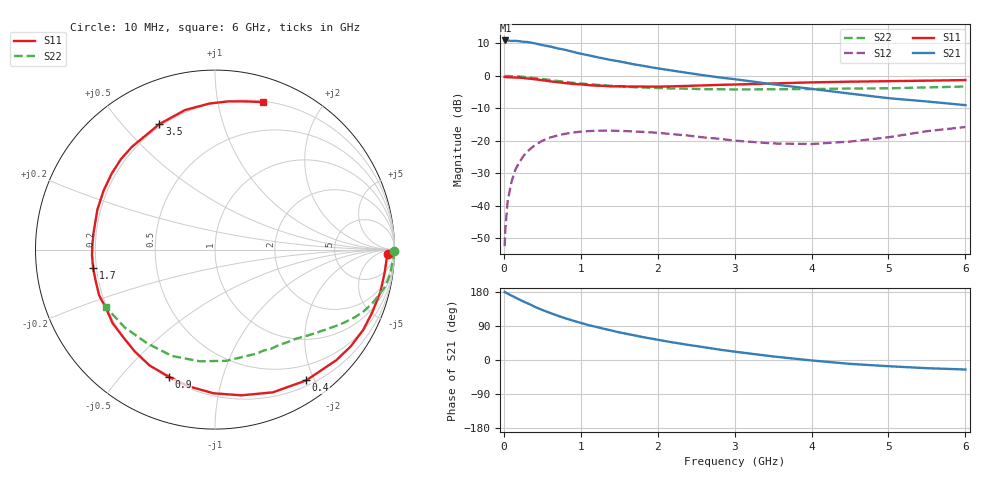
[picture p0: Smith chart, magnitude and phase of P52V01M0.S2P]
! SIEMENS Small Signal Semiconductors
! BFP183
! Si NPN RF Bipolar Junction Transistor in SOT143
! VCE = 2 V  IC = 1 mA
! Common Emitter S-Parameters:  March  1996
# GHz  S  MA  R  50
!  f  S11  S21  S12  S22
! GHz  MAG  ANG  MAG  ANG  MAG  ANG  MAG  ANG
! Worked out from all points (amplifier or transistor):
!   36 points, 10 MHz to 6 GHz, reference 50 ohm
!   highest |S21| = 10.9 dB at 20 MHz (marker M1)
!   |S21| within 3 dB of that: start of sweep to 816.7 MHz
!   unconditionally stable (mu >= 1): 2.458 GHz to end of sweep
!   at 250 MHz: K = 0.10, MSG = 17.7 dB, |S12| = -24.8 dB
!   at 1.4 GHz: K = 0.55, MSG = 10.9 dB, |S12| = -16.8 dB
!   at 6 GHz: K = 1.06, MAG = 1.9 dB, |S12| = -15.7 dB
!   S11 on the Smith chart (normalised r, x): 10 MHz: 37, -24; 400 MHz: 0.27, -1.89; 900 MHz: 0.21, -0.68; 1.7 GHz: 0.19, -0.07; 3.5 GHz: 0.19, +0.63; 6 GHz: 0.21, +1.35
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0.01  0.9625 -1.4  3.472 179.4  0.0024 83.9  0.9999 -0.5
0.02  0.958 -2.9  3.51 178.6  0.0045 84.9  0.9914 -1.0
0.05  0.9543 -7.3  3.505 175.1  0.0119 88.8  0.9961 -2.5
0.1  0.9514 -14.3  3.447 170.0  0.0236 80.3  0.9894 -5.0
0.15  0.9432 -21.8  3.464 164.8  0.0359 76.4  0.9858 -7.7
0.2  0.9392 -28.4  3.416 159.7  0.0466 72.6  0.9781 -10.1
0.3  0.9148 -42.3  3.329 150.5  0.0677 64.6  0.9537 -14.6
0.4  0.8884 -55.1  3.172 140.6  0.0855 56.9  0.9264 -18.9
0.5  0.8583 -67.9  2.977 131.9  0.1005 49.7  0.8965 -22.6
0.6  0.8251 -79.7  2.838 124.3  0.1126 43.6  0.8659 -25.8
0.7  0.8006 -90.6  2.65 116.9  0.1214 37.7  0.8346 -28.7
0.8  0.7755 -101.1  2.514 110.0  0.1288 32.5  0.8088 -31.2
0.9  0.7533 -110.1  2.345 103.8  0.1345 27.8  0.7835 -33.5
1.1  0.7222 -128.4  2.077 92.2  0.1415 19.7  0.745 -37.5
1.4  0.6898 -151.2  1.751 77.8  0.1438 9.8  0.7034 -43.0
1.7  0.687 -171.3  1.501 64.9  0.1392 2.9  0.669 -48.1
2.2  0.692 161.3  1.202 46.3  0.1267 -4.8  0.6392 -56.6
2.8  0.7271 136.2  0.948 27.5  0.1078 -7.9  0.6243 -68.3
3.5  0.7648 113.9  0.743 9.4  0.0913 -0.7  0.6229 -84.2
4.5  0.8144 92.2  0.534 -10.2  0.0976 18.0  0.6393 -112.1
5.5  0.8442 77.9  0.404 -21.6  0.1411 25.1  0.6644 -139.3
6  0.8636 72.1  0.355 -25.1  0.1635 22.4  0.6865 -152.0
